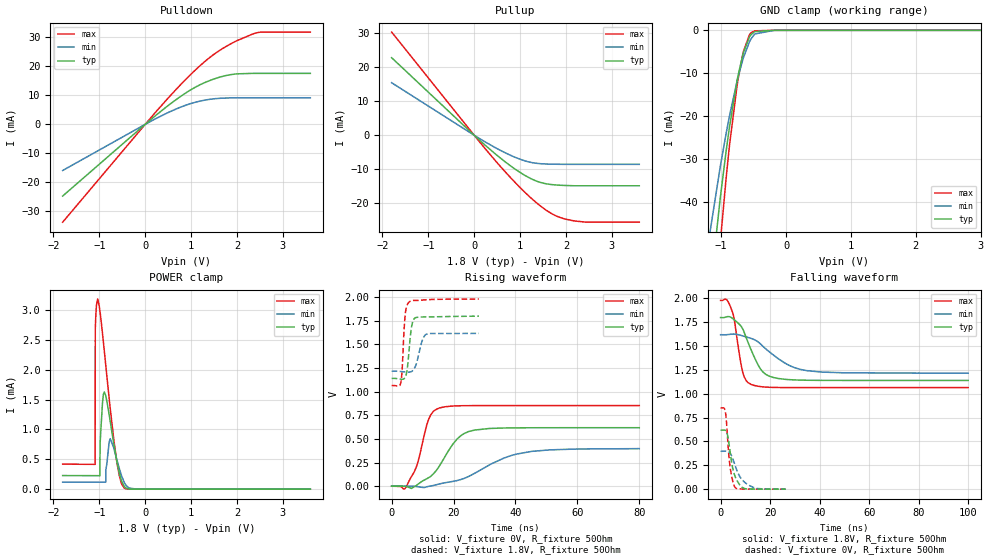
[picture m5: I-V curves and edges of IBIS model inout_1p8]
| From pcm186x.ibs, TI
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|   inout_1p8 Model
[Model]   inout_1p8
Model_type   I/O
Polarity   Non-Inverting
Enable   Active-High
Vinl = 0.54
Vinh = 1.26
Vmeas = 0.9
Vref = 0
Cref = 20pF
Rref = 200
|   typ   min   max
|   (nom PVT)   (fast PVT)   (slow PVT)
C_comp   6.641e-12   6.126e-12   6.887e-12
[Model spec]
|subparameter
Vinl   0.54   0.486   0.594
Vinh   1.26   1.134   1.386
| Where nom  PVT is Nominal Process, 1.8V, 27C
|   Fast PVT is Strong Process,  1.98V, -40C
|   Slow PVT is Weak Process,   1.62V, 125C
[Voltage Range]   1.8   1.62   1.98
|Junction Temperature
[Temperature Range]   27   125   -40
[Pullup Reference]   1.8   1.62   1.98
[Pulldown Reference]   0   0   0
[Power Clamp Reference]   1.8   1.62   1.98
[GND Clamp Reference]   0   0   0
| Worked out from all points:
|   slope of the pulldown table from 0 to 0.27 V, typ, clamps not added: 75.4 ohm
|   slope of the pullup table from 0 to 0.27 V, typ, clamps not added: 82.2 ohm
|   GND clamp passes 1 mA (typ) near -0.54 V on its own axis
|   POWER clamp passes 1 mA (typ) near -0.74 V on its own axis
|   falling waveform, V_fixture 1.8V, R_fixture 50Ohm: 20-80 % time 6.67ns typ, 12.4ns min, 3.36ns max; typ from 1.8 V to 1.14 V
|   rising waveform, V_fixture 0V, R_fixture 50Ohm: 20-80 % time 7.78ns typ, 14.9ns min, 4.12ns max; typ from 0 V to 0.619 V
|   rising waveform, V_fixture 1.8V, R_fixture 50Ohm: 20-80 % time 1.19ns typ, 1.86ns min, 923ps max; typ from 1.14 V to 1.8 V
|   falling waveform, V_fixture 0V, R_fixture 50Ohm: 20-80 % time 2.72ns typ, 4.48ns min, 1.79ns max; typ from 0.619 V to 0 V
[Pulldown]
|   Voltage   I(typ)   I(min)   I(max)
-1.8V     -24.7mA    -15.9mA    -33.71mA
37.08mV   503.6uA    322.1uA    691.2uA
469.1mV   6.093mA    3.831mA    8.506mA
977.9mV   11.73mA    7.081mA    16.96mA
1.205V    13.71mA    8.034mA    20.33mA
1.44V     15.29mA    8.69mA     23.42mA
1.867V    17.12mA    9.107mA    27.74mA
2.43V     17.55mA    9.135mA    31.52mA
2.512V    17.55mA    9.135mA    31.77mA
3.6V      17.55mA    9.135mA    31.77mA
[GND Clamp]
|   Voltage   I(typ)   I(min)   I(max)
-1.8V     -274mA     -172mA     -383.3mA
-1.162V   -59.61mA   -45.98mA   -78.12mA
-1.013V   -38.93mA   -31.66mA   -49.29mA
-925.2mV  -28.28mA   -24.11mA   -34.63mA
-869.4mV  -22.23mA   -19.73mA   -26.46mA
-736.2mV  -10.28mA   -10.66mA   -11.09mA
-657.5mV  -5.238mA   -6.396mA   -4.955mA
-564.5mV  -1.563mA   -2.689mA   -1.03mA
-538.2mV  -983.7uA   -1.952mA   -555.3uA
-481.3mV  -292.5uA   -842.1uA   -114uA
-180mV    -19.95nA   -834.7nA   0A
3.6V      0A         0A         0A
[Pullup]
|   Voltage   I(typ)   I(min)   I(max)
-1.8V     22.81mA    15.44mA    30.34mA
0V        0A         0A         0A
469.1mV   -5.583mA   -3.716mA   -7.59mA
787.1mV   -8.952mA   -5.87mA    -12.38mA
1.033V    -11.22mA   -7.214mA   -15.82mA
1.267V    -12.96mA   -8.068mA   -18.8mA
1.438V    -13.85mA   -8.36mA    -20.74mA
1.604V    -14.36mA   -8.477mA   -22.35mA
1.788V    -14.64mA   -8.53mA    -23.74mA
2.179V    -14.86mA   -8.559mA   -25.2mA
2.449V    -14.86mA   -8.559mA   -25.57mA
3.6V      -14.86mA   -8.559mA   -25.57mA
[POWER Clamp]
|   Voltage   I(typ)   I(min)   I(max)
-1.8V     227.8uA    118.2uA    419.5uA
-1.091V   226uA      117.3uA    415.4uA
-1.089V   226uA      117.3uA    2.681mA
-1.038V   225.9uA    117.3uA    3.185mA
-986.4mV  225.4uA    117.2uA    2.98mA
-984.6mV  748.5uA    117.2uA    2.969mA
-930.1mV  1.461mA    117.1uA    2.598mA
-891mV    1.627mA    117uA      2.308mA
-763.2mV  1.135mA    844.9uA    1.356mA
-615.6mV  454.2uA    485.5uA    440.5uA
-459.5mV  48.16uA    118.2uA    21.74uA
3.6V      0A         0A         0A
[Ramp]
R_load = 50
|   typ   min   max
dV/dt_r   0.371256/7.75981e-09   0.238396/1.48443e-08   0.511668/4.10345e-09
dV/dt_f   0.395729/6.65952e-09   0.242168/1.23792e-08   0.548784/3.33475e-09
[Falling Waveform]
V_fixture = 1.8V
V_fixture_min = 1.62V
V_fixture_max = 1.98V
R_fixture = 50Ohm
|   Time   V(typ)   V(min)   V(max)
0s        1.8V       1.62V      1.98V
2.47ns    1.808V     1.62V      1.987V
4.72ns    1.793V     1.627V     1.863V
8.96ns    1.68V      1.607V     1.225V
12.42ns   1.456V     1.58V      1.097V
17.14ns   1.229V     1.497V     1.073V
23.48ns   1.16V      1.365V     1.066V
30.03ns   1.146V     1.273V     1.065V
40.93ns   1.141V     1.228V     1.065V
100ns     1.14V      1.216V     1.065V
[Rising Waveform]
V_fixture = 0V
V_fixture_min = 0V
V_fixture_max = 0V
R_fixture = 50Ohm
|   Time   V(typ)   V(min)   V(max)
0s        502.9pV    41.48nV    283.2pV
4.68ns    -3.362mV   161.3uV    -7.219mV
8.18ns    12.37mV    -4.436mV   222.7mV
12.09ns   93.1mV     -1.525mV   717.3mV
15.43ns   213.6mV    23.64mV    827.3mV
21.24ns   501.6mV    60.18mV    850.2mV
26.89ns   594.4mV    137.4mV    852.5mV
36.25ns   615.7mV    297.2mV    852.7mV
45.26ns   618.2mV    368.3mV    852.8mV
79.98ns   618.8mV    397.3mV    852.8mV
[Rising Waveform]
V_fixture = 1.8V
V_fixture_min = 1.62V
V_fixture_max = 1.98V
R_fixture = 50Ohm
|   Time   V(typ)   V(min)   V(max)
0s        1.14V      1.216V     1.065V
2.93ns    1.132V     1.214V     1.089V
3.34ns    1.131V     1.212V     1.206V
4.39ns    1.152V     1.209V     1.814V
4.87ns    1.204V     1.207V     1.905V
5.61ns    1.426V     1.207V     1.947V
6.45ns    1.688V     1.213V     1.962V
7.45ns    1.778V     1.252V     1.965V
11ns      1.792V     1.605V     1.972V
28.18ns   1.799V     1.616V     1.98V
[Falling Waveform]
V_fixture = 0V
V_fixture_min = 0V
V_fixture_max = 0V
R_fixture = 50Ohm
|   Time   V(typ)   V(min)   V(max)
0s        618.8mV    397.3mV    852.8mV
1.95ns    617mV      398.7mV    809.1mV
2.35ns    603.8mV    399.1mV    717.1mV
2.82ns    565.6mV    397.6mV    537.5mV
3.75ns    409.9mV    380.9mV    253mV
4.94ns    215.7mV    317.1mV    82.38mV
5.98ns    126.1mV    240.2mV    14.96mV
8.61ns    20.27mV    100.5mV    1.754mV
13.27ns   1.368mV    17.94mV    293.3uV
26.26ns   54.25uV    445.8uV    -1.973uV
